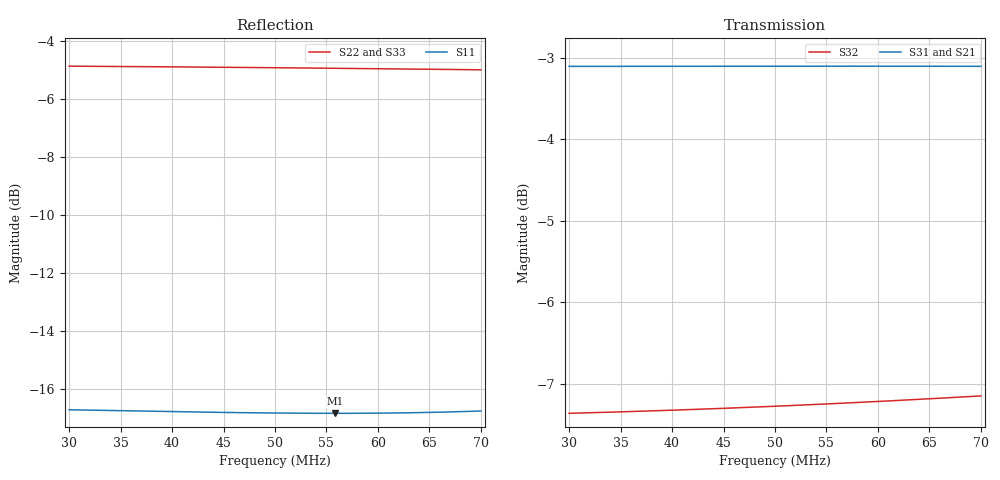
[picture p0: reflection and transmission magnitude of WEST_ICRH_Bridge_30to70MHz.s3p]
! Touchstone file exported from HFSS 2020.2.0
!  File:  C:/Users/JH218595/Documents/ICRH/WEST/HFSS_antenna_elements/Bridge_ImpTrasnf_Stub.aedt
!  Generated:  5:41:10  juil. 31, 2020
!  Design:  Bridge
!  Project:  Bridge_ImpTrasnf_Stub
!  Setup:  Setup1
!  Solution:  Sweep_operationnal
!Data is not renormalized
# GHZ S MA
! Terminal data exported
! Port[1] = 1
! Port[2] = 2
! Port[3] = 3
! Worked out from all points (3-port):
!   4001 points, 30 MHz to 70 MHz, reference per port
!   strongest paths, dB at 30 MHz, 40 MHz, 50 MHz, 60 MHz, 70 MHz:
!     S31: -3.1, -3.1, -3.1, -3.1, -3.1
!     S21: -3.1, -3.1, -3.1, -3.1, -3.1
!     S32: -7.4, -7.3, -7.3, -7.2, -7.2
!   lowest |S11| = -16.8 dB at 55.86 MHz (marker M1), VSWR 1.34
!   |S11| at or under -10 dB: start of sweep to end of sweep
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0.03  0.1461 -28.2  0.6994 -14.2  0.6994 -14.1
      0.6994 -14.2  0.572 170.6  0.4283 -12.6
      0.6994 -14.1  0.4283 -12.6  0.572 170.7
0.0348  0.1455 -33.0  0.6995 -16.4  0.6995 -16.4
        0.6995 -16.4  0.5713 169.2  0.4292 -14.6
        0.6995 -16.4  0.4292 -14.6  0.5713 169.2
0.03992  0.145 -38.3  0.6995 -18.9  0.6995 -18.8
         0.6995 -18.9  0.5705 167.6  0.4302 -16.8
         0.6995 -18.8  0.4302 -16.8  0.5704 167.6
0.04496  0.1445 -43.6  0.6995 -21.3  0.6996 -21.2
         0.6995 -21.3  0.5695 166.1  0.4313 -18.9
         0.6996 -21.2  0.4313 -18.9  0.5695 166.1
0.05  0.1442 -49.0  0.6996 -23.7  0.6996 -23.6
      0.6996 -23.7  0.5685 164.5  0.4326 -21.1
      0.6996 -23.6  0.4326 -21.1  0.5685 164.6
0.05586  0.144 -55.5  0.6996 -26.5  0.6996 -26.4
         0.6996 -26.5  0.5672 162.8  0.4343 -23.7
         0.6996 -26.4  0.4343 -23.7  0.5672 162.8
0.05953  0.1441 -59.7  0.6996 -28.2  0.6996 -28.2
         0.6996 -28.2  0.5664 161.7  0.4354 -25.3
         0.6996 -28.2  0.4354 -25.3  0.5663 161.8
0.0632  0.1443 -64.0  0.6995 -30.0  0.6996 -30.0
        0.6995 -30.0  0.5655 160.6  0.4366 -26.9
        0.6996 -30.0  0.4366 -26.9  0.5654 160.7
0.06814  0.145 -69.9  0.6995 -32.4  0.6995 -32.3
         0.6995 -32.4  0.5643 159.2  0.4383 -29.2
         0.6995 -32.3  0.4383 -29.2  0.5642 159.3
0.07  0.1453 -72.2  0.6994 -33.3  0.6995 -33.2
      0.6994 -33.3  0.5638 158.7  0.439 -30.0
      0.6995 -33.2  0.439 -30.0  0.5637 158.7
